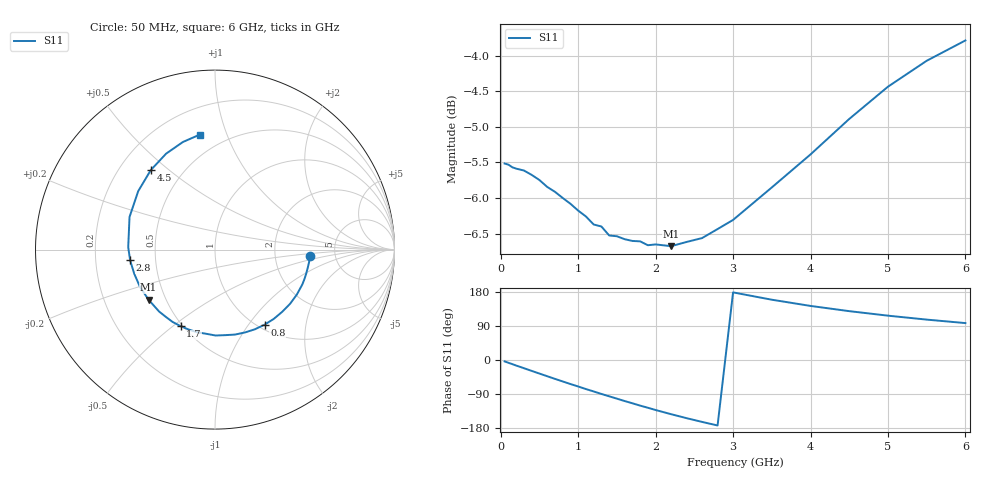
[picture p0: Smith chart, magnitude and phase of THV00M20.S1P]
! SIEMENS Discrete & RF Semiconductors
! BAS70
! Si Schottky Diode in SOT23
! IF = 0.2 mA
! S-Parameters:  February  1997
# GHz  S  MA  R  50
!  f  S11
! GHz  MAG  ANG
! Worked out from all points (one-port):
!   34 points, 50 MHz to 6 GHz, reference 50 ohm
!   lowest |S11| = -6.7 dB at 2.2 GHz (marker M1), VSWR 2.73, Z = 20.1 - j14.3 ohm
!   |S11| at or under -10 dB: nowhere
!   S11 on the Smith chart (normalised r, x): 50 MHz: 3.22, -0.31; 800 MHz: 1.07, -1.20; 1.7 GHz: 0.49, -0.53; 2.8 GHz: 0.36, -0.05; 4.5 GHz: 0.33, +0.43; 6 GHz: 0.37, +0.81
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0.05  0.5299 -3.7
0.15  0.5266 -10.9
0.25  0.5247 -18.1
0.4  0.5202 -28.8
0.5  0.5159 -35.8
0.6  0.5102 -42.8
0.7  0.5062 -49.8
0.8  0.5012 -56.6
0.9  0.4965 -63.4
1.1  0.4864 -76.7
1.3  0.4786 -89.6
1.4  0.4717 -95.8
1.5  0.4711 -102.0
1.6  0.4688 -108.3
1.7  0.4675 -114.2
1.8  0.4672 -120.4
2  0.4649 -132.0
2.2  0.4636 -143.0
2.4  0.4667 -153.5
2.6  0.4697 -163.4
2.8  0.4766 -172.8
3  0.4837 178.4
3.5  0.5098 159.1
4  0.5377 142.7
4.5  0.5695 128.9
5  0.5999 117.0
5.5  0.6256 106.6
6  0.6465 97.4
